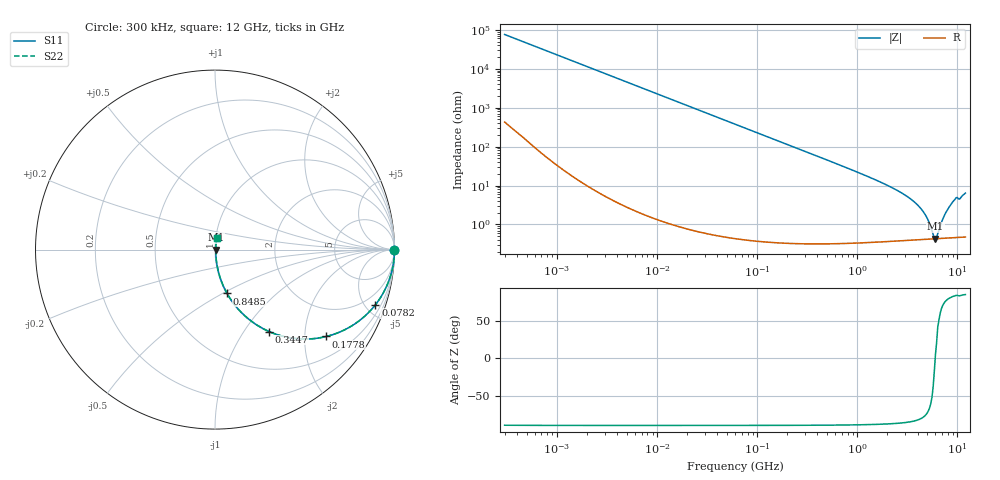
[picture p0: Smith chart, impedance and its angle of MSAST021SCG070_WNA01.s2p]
! MSAST021SCG070_WNA01  S-PARAMETER MODEL  ( General Type )
! Model Generated by TAIYO YUDEN Corporation (http://www.ty-top.com)
! Version 2.0
! TAIYO YUDEN Control No. 181101
! Copyright(c) 2015 TAIYO YUDEN CO.,LTD. All Rights Reserved.
! Product Description (link to TY-COMPAS)
! https://ds.yuden.co.jp/TYCOMPAS/or/detail?pn=MSAST021SCG070CWNA01&u=M
! Products Name : Multilayer Ceramic Capacitors
! Characteristics :
!  Capacitance : 7 pF , Rated Voltage : 25V , TCC : CG / C0G
!  Case Size : 0.25 x 0.125 / 0.0098 x 0.0049 [mm/inch] , Thickness : 0.125 / 0.0049 [mm/inch]
!  (Conditions: Temperature = 25 degC , DC Bias Current/Voltage = 0A / 0V)
! External Node Assignments :
!  1  o---| |---o  2
! GND o---------o GND
! Frequency Range : 0.3MHz  -  12000MHz  [ 401 STEP ]
# MHz S RI R 50
! Freq[MHz].  S11 Real  S11 Imag  S21 Real  S21 Imag  S12 Real  S12 Imag  S22 Real  S22 Imag
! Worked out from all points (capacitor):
!   401 points, 300 kHz to 12 GHz, reference 50 ohm
!   read as one part in series: C = 7 pF near 316.3 kHz
!   lowest |Z| = 433 mohm at 6.026 GHz (marker M1)
!   series resonance near 5.994 GHz, so ESL is about 100 pH
!   S11 on the Smith chart (normalised r, x): 300 kHz: open; 78.2 MHz: 1.01, -5.81; 177.8 MHz: 1.01, -2.56; 344.7 MHz: 1.01, -1.31; 848.5 MHz: 1.01, -0.53; 12 GHz: 1.01, +0.13
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0.3  1 -0.00132  9.18e-06 0.00132  9.18e-06 0.00132  1 -0.00132
1.769972  0.9999 -0.00778  6.78e-05 0.00778  6.78e-05 0.00778  0.9999 -0.00778
10.44266  0.9979 -0.0458  0.00213 0.0458  0.00213 0.0458  0.9979 -0.0458
27.10171  0.9859 -0.1175  0.0141 0.1175  0.0141 0.1175  0.9859 -0.1175
60  0.9346 -0.2466  0.0654 0.2466  0.0654 0.2466  0.9346 -0.2466
78.19928  0.8939 -0.3073  0.1061 0.3073  0.1061 0.3073  0.8939 -0.3073
177.7716  0.6199 -0.4841  0.3801 0.4841  0.3801 0.4841  0.6199 -0.4841
344.7396  0.3026 -0.457  0.6974 0.457  0.6974 0.457  0.3026 -0.457
353.9943  0.2915 -0.452  0.7085 0.452  0.7085 0.452  0.2915 -0.452
540.8523  0.15 -0.3533  0.85 0.3533  0.85 0.3533  0.15 -0.3533
848.5281  0.0672 -0.2441  0.9328 0.2441  0.9328 0.2441  0.0672 -0.2441
2088.533  0.0126 -0.094  0.9874 0.094  0.9874 0.094  0.0126 -0.094
3190.978  0.00645 -0.0504  0.9935 0.0504  0.9935 0.0504  0.00645 -0.0504
4158.869  0.00484 -0.0279  0.9952 0.0279  0.9952 0.0279  0.00484 -0.0279
4875.354  0.0044 -0.0155  0.9956 0.0155  0.9956 0.0155  0.0044 -0.0155
5715.274  0.00427 -0.00338  0.9957 0.00338  0.9957 0.00338  0.00427 -0.00338
6026.253  0.00429 0.000359  0.9957 -0.000359  0.9957 -0.000359  0.00429 0.000359
6354.153  0.00434 0.00388  0.9957 -0.00388  0.9957 -0.00388  0.00434 0.00388
7448.838  0.00472 0.0169  0.9953 -0.0169  0.9953 -0.0169  0.00472 0.0169
8503.825  0.00545 0.0305  0.9945 -0.0305  0.9945 -0.0305  0.00545 0.0305
9454.42  0.00649 0.0435  0.9935 -0.0435  0.9935 -0.0435  0.00649 0.0435
12000  0.00873 0.0629  0.9913 -0.0629  0.9913 -0.0629  0.00873 0.0629
